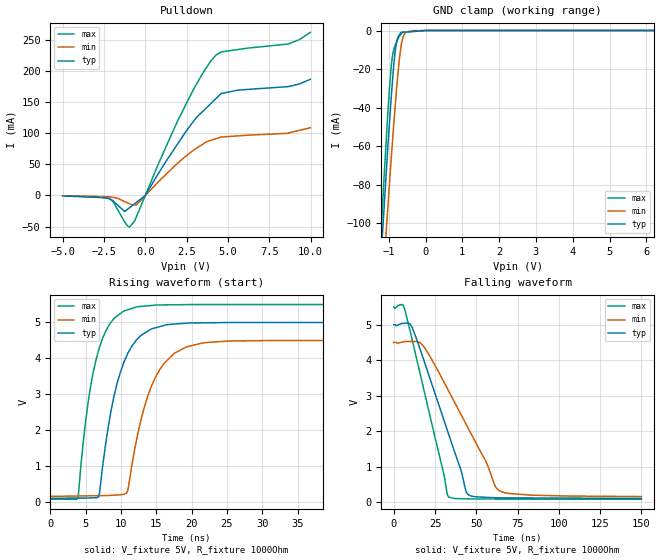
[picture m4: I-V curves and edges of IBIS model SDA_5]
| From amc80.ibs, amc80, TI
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[Model]  SDA_5
Model_type   I/O_open_drain
Polarity   Non-Inverting
Enable   Active-Low
Vinl = 0.8
Vinh = 2
Vmeas = 2.5
Vref = 2.5
Cref = 15pF
Rref = 50
|   typ   min   max
|   (nom PVT)   (Fast PVT)   (slow PVT)
|   BUFFER OUTPUT TURNED HIGH or as an INPUT
|C_comp   1.175E-12   9.956E-13   1.393E-12
|   BUFFER OUTPUT TURNED LOW
C_comp   8.711E-13   8.552E-13   9.249E-13
| Where   nom PVT is  Nominal Process, 5.0V, 27C
|   Fast PVT is Strong Process, 5.5V, -40C
|   Slow PVT is Weak Process, 4.5V, 125C
|C_comp - from L-C Tank method, L = 1nH, peak frequency
[Voltage Range]   5   4.5   5.5
[Temperature Range]   27   125   -40
[Pullup Reference]   5   4.5   5.5
[Pulldown Reference]   0   0   0
[Power Clamp Reference]   5   4.5   5.5
[GND Clamp Reference]   0   0   0
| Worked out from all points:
|   slope of the pulldown table from 0 to 0.75 V, typ, clamps not added: 22.6 ohm
|   GND clamp passes 1 mA (typ) near -0.67 V on its own axis
|   falling waveform, V_fixture 5V, R_fixture 1000Ohm: 20-80 % time 21.3ns typ, 29.3ns min, 16.5ns max; typ from 5 V to 0.109 V
|   rising waveform, V_fixture 5V, R_fixture 1000Ohm: 20-80 % time 3.23ns typ, 3.79ns min, 2.74ns max; typ from 0.109 V to 5 V
[Pulldown]
|   Voltage   I(typ)   I(min)   I(max)
-5V       -736.2uA   -519.2uA   -724.3uA
-2.165V   -5.561mA   -2.16mA    -4.932mA
-1.246V   -25.73mA   -9.848mA   -42.54mA
-960.7mV  -19.83mA   -13.15mA   -50.82mA
-536.6mV  -11.07mA   -14.91mA   -34.08mA
997.3uV   45.34uA    22.92uA    64.51uA
1.976V    83.43mA    52.11mA    120.6mA
3.416V    133.3mA    81.18mA    193.2mA
4.279V    155.5mA    91.16mA    225.2mA
5.561V    168.7mA    95.48mA    233.9mA
8.631V    174.5mA    100mA      242.9mA
9.985V    186.3mA    108.6mA    261.6mA
[GND Clamp]
|   Voltage   I(typ)   I(min)   I(max)
-5V       -1.389A    -1.299A    -1.55A
-1.233V   -125.2mA   -150.7mA   -114mA
-1.129V   -93.06mA   -121.4mA   -77.29mA
-1.046V   -67.42mA   -97.98mA   -49.6mA
-978.9mV  -47.73mA   -79.13mA   -29.76mA
-918.4mV  -31.38mA   -62.93mA   -16.22mA
-853.1mV  -16mA      -46mA      -9.318mA
-786.6mV  -6.074mA   -30.26mA   -6.005mA
-666.3mV  -1.001mA   -8.45mA    -1.877mA
-551.3mV  -828.5uA   -1.033mA   -749.4uA
-348.9mV  -525uA     -5.75uA    -463.2uA
9.985V    0A         0A         0A
[POWER Clamp]
|   SCR cell for ESD function. Effects occurr above VDD x 2
|   Voltage   I(typ)   I(min)   I(max)
-5V       0A         0A         0A
0V        0A         0A         0A
10V       0A         0A         0A
[Ramp]
R_load = 1000
|   typ   min   max
dV/dt_r   2.93445/3.22272e-009   2.60322/3.77716e-009   3.25023/2.73267e-009
dV/dt_f   2.93445/2.12615e-008   2.60322/2.93646e-008   3.25022/1.64412e-008
[Falling Waveform]
V_fixture = 5V
V_fixture_min = 4.5V
V_fixture_max = 5.5V
R_fixture = 1000Ohm
C_fixture = 0F
|   Time   V(typ)   V(min)   V(max)
0s        5V         4.5V       5.5V
6.489ns   5.04V      4.523V     5.464V
10.03ns   5.016V     4.526V     4.797V
16.27ns   4.27V      4.483V     3.562V
30.4ns    2.312V     3.386V     781.1mV
32.34ns   2.042V     3.214V     241mV
33.39ns   1.895V     3.121V     148.1mV
44.35ns   254.7mV    2.153V     95.87mV
64.17ns   125.2mV    319.7mV    89.58mV
150ns     109.2mV    161.3mV    82.96mV
[Rising Waveform]
V_fixture = 5V
V_fixture_min = 4.5V
V_fixture_max = 5.5V
R_fixture = 1000Ohm
C_fixture = 0F
|   Time   V(typ)   V(min)   V(max)
0s        109.2mV    161.3mV    82.95mV
3.906ns   114.1mV    172.8mV    111.1mV
5.334ns   115.9mV    177mV      2.748V
6.848ns   155.6mV    181.4mV    4.229V
8.637ns   2.581V     192mV      5.015V
10.79ns   4.06V      254.8mV    5.341V
12.22ns   4.519V     1.751V     5.433V
16.13ns   4.919V     3.87V      5.488V
21.96ns   4.991V     4.44V      5.499V
150ns     5V         4.5V       5.5V
